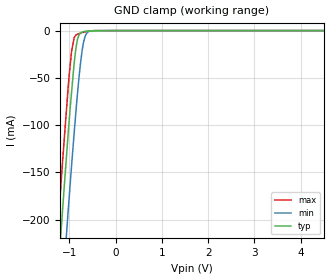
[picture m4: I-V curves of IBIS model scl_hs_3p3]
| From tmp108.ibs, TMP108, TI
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|   scl_hs_3p3 Model
[Model]   scl_hs_3p3
Model_type   Input
Vinl = 0.5
Vinh = 1.4
|   typ   min   max
C_comp   2.619e-13   2.608e-13   2.635e-13
| Where nom  PVT is Nominal Process, 3.3V, 27C
|   Fast PVT is Strong Process,  3.6V, -40C
|   Slow PVT is Weak Process,   3V, 125C
[Voltage Range]   3.3   3   3.6
|Ambient Temperature   25   125   -40
|Junction Temperature
[Temperature Range]   27   125   -40
[Power Clamp Reference]   3.3   3   3.6
[GND Clamp Reference]   0   0   0
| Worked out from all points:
|   GND clamp passes 1 mA (typ) near -0.68 V on its own axis
[GND Clamp]
|   Voltage   I(typ)   I(min)   I(max)
-3.3V     -1.779A    -1.848A    -1.738A
-1.27V    -275.6mA   -358.8mA   -225.2mA
-1.152V   -192.8mA   -275.9mA   -141.6mA
-1.099V   -156.7mA   -239.9mA   -106.9mA
-1.03V    -111mA     -193mA     -61.73mA
-954mV    -65.81mA   -143.6mA   -22.28mA
-896.4mV  -34.16mA   -107.7mA   -7.352mA
-828.3mV  -9.983mA   -68.34mA   -3.962mA
-726mV    -1.598mA   -21.56mA   -2.217mA
-624mV    -532.7uA   -2.624mA   -960.3uA
-468mV    -381uA     -82.81uA   -49.82uA
6.6V      0A         0A         0A
[POWER Clamp]
|   Voltage   I(typ)   I(min)   I(max)
-3.3V     0A         0A         0A
-3.298V   0A         0A         0A
6.6V      0A         0A         0A
